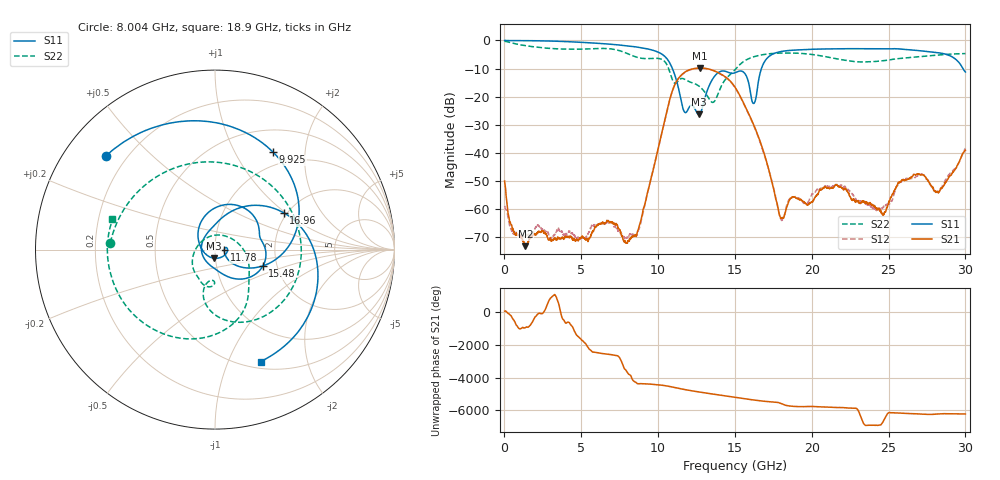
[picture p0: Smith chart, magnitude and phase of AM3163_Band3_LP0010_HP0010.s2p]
!Agilent Technologies,E8364B,MY43040894,A.07.50.67
!Agilent E8364B: A.07.50.67
!Date: Thursday, August 20, 2020 11:05:05
!Correction: S11(Full 2 Port(1,2))
!S21(Full 2 Port(1,2))
!S12(Full 2 Port(1,2))
!S22(Full 2 Port(1,2))
!S2P File: Measurements: S11, S21, S12, S22:
# Hz S  dB  R 50
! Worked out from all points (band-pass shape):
!   3201 points, 10 MHz to 30 GHz, reference 50 ohm
!   highest |S21| = -9.83 dB at 12.74 GHz (marker M1); lowest = -73.3 dB at 1.369 GHz (marker M2)
!   |S21| within 3 dB of the highest: 11.43 GHz to 14.34 GHz (2.913 GHz wide, 22.6 % of centre)
!   lowest |S11| = -26.3 dB at 12.64 GHz (marker M3), VSWR 1.10, Z = 49 - j4.69 ohm
!   |S11| at or under -10 dB: 10.93 GHz to 16.73 GHz (5.794 GHz wide, 41.9 % of centre); 29.84 GHz to end of sweep
!   |S22| runs from -22.1 to -0.3 dB; largest |S21 - S12| = 0.0041
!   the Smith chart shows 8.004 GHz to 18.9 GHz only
!   S11 on the Smith chart (normalised r, x): 8.004 GHz: 0.13, +0.37; 9.925 GHz: 0.80, +1.44; 11.78 GHz: 1.11, -0.01; 15.48 GHz: 1.68, -0.34; 16.96 GHz: 1.92, +0.97; 18.9 GHz: 0.58, -1.32
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1e7  0.00 -1.9  -50.06 75.3  -58.95 95.1  -0.27 -6.9
1.368922e9  -0.06 -37.5  -73.29 152.7  -69.83 77.2  -1.86 -113.9
2.755959e9  -0.18 -75.3  -69.38 48.5  -68.22 -79.6  -2.75 163.4
5.014581e9  -0.67 -135.3  -70.01 100.1  -70.43 94.2  -3.09 44.0
6.851469e9  -1.33 174.6  -64.92 -58.3  -64.36 -61.5  -2.96 -78.5
8.004209e9  -1.92 139.4  -72.21 -87.8  -70.00 135.5  -4.67 176.3
8.847678e9  -2.53 109.3  -64.72 -56.3  -65.66 -59.3  -6.27 86.4
9.925444e9  -3.98 59.2  -40.34 -117.4  -40.45 -118.9  -6.35 -22.9
1.000979e10  -4.18 54.2  -38.39 -125.5  -38.51 -127.1  -6.40 -31.1
1.178108e10  -25.70 -2.9  -11.15 -66.3  -11.26 -66.2  -13.97 -111.7
1.264329e10  -26.31 -99.3  -9.84 156.7  -9.90 157.1  -16.19 -143.4
1.273701e10  -25.92 -128.0  -9.83 143.0  -9.87 143.4  -16.59 -148.5
1.5005e10  -11.51 9.8  -16.63 -179.1  -16.81 -179.0  -10.43 -51.5
1.548297e10  -11.01 -19.4  -21.39 113.5  -21.58 114.0  -7.83 -71.7
1.623272e10  -22.43 -176.6  -30.17 19.8  -30.47 20.1  -5.80 -104.1
1.696372e10  -7.24 28.2  -41.41 -62.3  -41.75 -58.9  -4.94 -131.3
1.801337e10  -3.93 -34.8  -63.48 166.5  -63.80 -178.8  -4.48 -166.8
1.89037e10  -3.42 -67.7  -55.83 -15.1  -55.66 -11.1  -4.50 163.4
2.000958e10  -3.14 -99.0  -57.43 -13.6  -54.84 -16.7  -4.98 123.6
2.25025e10  -2.93 -157.2  -55.65 -116.7  -53.74 -123.6  -7.34 12.2
2.500479e10  -2.99 145.2  -58.11 -40.0  -58.28 -41.3  -6.97 -101.8
3e10  -11.25 -22.0  -39.10 -116.2  -38.37 -117.3  -4.68 100.9
